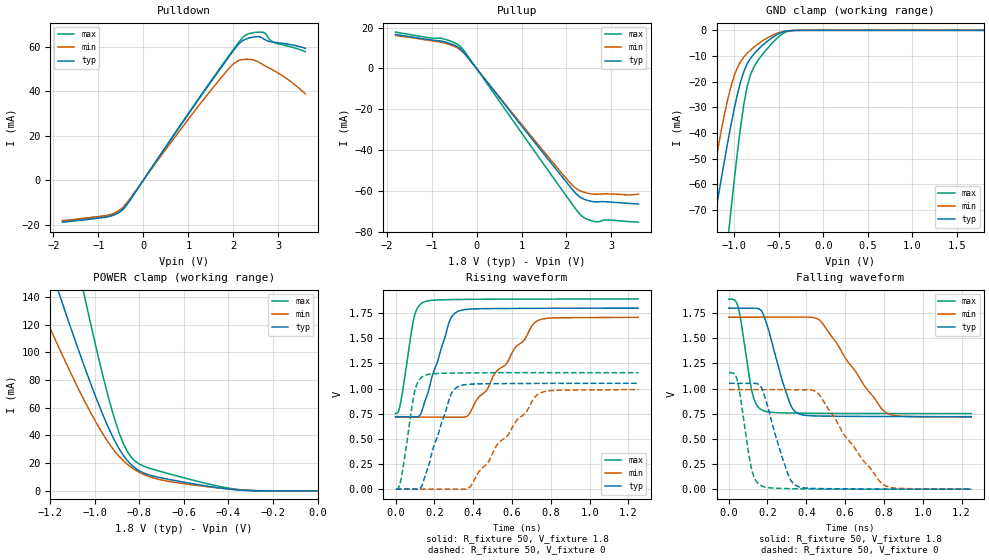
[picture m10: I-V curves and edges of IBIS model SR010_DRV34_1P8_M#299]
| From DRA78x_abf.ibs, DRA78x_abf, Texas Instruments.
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| Model based on original model for DDR_DIFFIOPB_V
|   Sub model SR010_DRV34_1P8
[model]   SR010_DRV34_1P8_M#299
|[Description]  [1.8V-I/O-X-X]
|   , ,
|[Input Load]
|[Output Drive]
|Voltage   1.8V
|Mode   I/O
Model_type   I/O
Polarity   Non-Inverting
Enable   Active-Low
Vinl =  0.775
Vinh =  1.025
Cref =  15.0000pF
Rref =  100.0000M
Vref =  0V
Vmeas =  0.9
C_comp   2p   2p   2p
[Model Spec]
Vinl   0.78   0.735   0.825
Vinh   1.02   0.975   1.065
[Receiver Thresholds]
Tslew_ac = 0.5n
Vth = 0.9
Vth_max = 0.945
Vth_min = 0.81
Vinh_ac = 0.2
Vinh_dc = 0.125
Vinl_ac = -0.2
Vinl_dc = -0.125
[Temperature Range]   25   125   -40
[Voltage Range]   1.8   1.71   1.89
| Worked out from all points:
|   slope of the pulldown table from 0 to 0.27 V, typ, clamps not added: 33.3 ohm
|   slope of the pullup table from 0 to 0.27 V, typ, clamps not added: 35.5 ohm
|   GND clamp passes 1 mA (typ) near -0.48 V on its own axis
|   POWER clamp passes 1 mA (typ) near -0.38 V on its own axis
|   rising waveform, R_fixture 50, V_fixture 1.8: 20-80 % time 101ps typ, 243ps min, 53.2ps max; typ from 0.721 V to 1.8 V
|   rising waveform, R_fixture 50, V_fixture 0: 20-80 % time 101ps typ, 241ps min, 53.2ps max; typ from 0 V to 1.05 V
|   falling waveform, R_fixture 50, V_fixture 1.8: 20-80 % time 94.6ps typ, 214ps min, 55.3ps max; typ from 1.8 V to 0.721 V
|   falling waveform, R_fixture 50, V_fixture 0: 20-80 % time 96.6ps typ, 219ps min, 54.7ps max; typ from 1.05 V to 0 V
[POWER_clamp]
-1.8V     464.6mA    344.4mA    740.8mA
-1.273V   197mA      143.3mA    314.4mA
-1.164V   144mA      104.2mA    229mA
-1.145V   135.3mA    97.86mA    215mA
-1.055V   93.25mA    67.59mA    146.5mA
-1.036V   85.18mA    61.89mA    133.3mA
-909.1mV  35.72mA    28.41mA    50.73mA
-872.7mV  25.87mA    21.94mA    34.5mA
-818.2mV  16.45mA    15.08mA    21.33mA
-690.9mV  9.084mA    7.592mA    13.42mA
-400mV    1.38mA     1.43mA     2.039mA
0V        227.3nA    761nA      1.176uA
[Pulldown]
-1.8V     -18.96mA   -18.25mA   -18.29mA
-818.2mV  -16.64mA   -15.93mA   -16.11mA
-600mV    -15.26mA   -14.42mA   -14.86mA
-436.4mV  -12.77mA   -11.85mA   -12.76mA
1.255V    37.14mA    34.14mA    37.53mA
1.855V    54.25mA    49.2mA     54.74mA
2.073V    60.22mA    53.41mA    60.8mA
2.291V    63.64mA    54.44mA    65.5mA
2.618V    64.32mA    52.48mA    66.68mA
2.727V    62.98mA    51.19mA    65.69mA
2.891V    62.13mA    49.45mA    62.08mA
3.6V      59.37mA    38.9mA     57.88mA
[Pullup]
-1.8V     16.66mA    16.14mA    17.84mA
-1.036V   14.05mA    13.69mA    15mA
-763.6mV  13.33mA    12.72mA    14.68mA
-490.9mV  11.4mA     10.78mA    12.65mA
-327.3mV  8.923mA    8.488mA    10.05mA
2.018V    -56.27mA   -54.56mA   -63.19mA
2.182V    -60.67mA   -58.29mA   -68.22mA
2.345V    -63.65mA   -60.35mA   -72.46mA
2.509V    -64.94mA   -61.33mA   -74.33mA
2.673V    -65.44mA   -61.69mA   -75.21mA
2.891V    -65.36mA   -61.45mA   -74.26mA
3.6V      -66.47mA   -61.61mA   -75.37mA
[GND_clamp]
-1.8V     -200.8mA   -187.9mA   -345.9mA
-1.327V   -95.75mA   -76.22mA   -171.1mA
-1.255V   -80.19mA   -60.47mA   -144.9mA
-1.218V   -72.53mA   -52.92mA   -131.9mA
-1.073V   -43.32mA   -26.59mA   -81.54mA
-1.036V   -36.61mA   -21.6mA    -69.55mA
-963.6mV  -24.61mA   -14.37mA   -47.01mA
-854.5mV  -12.98mA   -8.864mA   -21.66mA
-781.8mV  -9.263mA   -6.573mA   -14.36mA
-672.7mV  -5.498mA   -3.827mA   -8.897mA
-345.5mV  -48.81uA   -73.08uA   -79.37uA
1.8V      227.3nA    3.986uA    988nA
[Ramp]
dV/dt_f   0.647957/94.640072p 0.59676242/0.21402689n  0.6831801/55.297889p
dV/dt_r 0.63285444/0.10159097n 0.59531046/0.24136669n  0.6962006/53.228439p
R_load = 50
[Rising Waveform]
R_fixture = 50
V_fixture = 1.8
V_fixture_min = 1.71
V_fixture_max = 1.89
0s        720.8mV    716.7mV    752.8mV
25.2ps    720.4mV    716.6mV    852.1mV
95.22ps   720mV      716.6mV    1.707V
125ps     732.3mV    716.6mV    1.832V
144.3ps   832.3mV    716.6mV    1.859V
275.5ps   1.657V     716.5mV    1.884V
320.9ps   1.767V     715.4mV    1.886V
377.2ps   1.79V      740.6mV    1.887V
729.5ps   1.798V     1.672V     1.89V
1.25ns    1.8V       1.71V      1.89V
[Rising Waveform]
R_fixture = 50
V_fixture = 0
V_fixture_min = 0
V_fixture_max = 0
1.723ps   0V         0V         0V
32.03ps   0V         0V         138.9mV
98.8ps    0V         0V         974.3mV
146.1ps   96.14mV    0V         1.127V
278.8ps   911.3mV    0V         1.154V
324.6ps   1.021V     0V         1.155V
384.9ps   1.044V     25.07mV    1.156V
524.2ps   1.049V     443.6mV    1.158V
740.7ps   1.051V     950.9mV    1.158V
1.252ns   1.053V     990.1mV    1.159V
[Falling Waveform]
R_fixture = 50
V_fixture = 1.8
V_fixture_min = 1.71
V_fixture_max = 1.89
0s        1.8V       1.71V      1.89V
46.31ps   1.8V       1.71V      1.826V
122.2ps   1.8V       1.71V      953.1mV
143.2ps   1.799V     1.71V      840.5mV
173.4ps   1.76V      1.71V      784.7mV
309ps     884.6mV    1.71V      757.5mV
356.5ps   753.8mV    1.71V      756mV
476.3ps   726.9mV    1.666V     753.8mV
812.5ps   722.3mV    759.6mV    752mV
1.25ns    720.8mV    716.7mV    751.8mV
[Falling Waveform]
R_fixture = 50
V_fixture = 0
V_fixture_min = 0
V_fixture_max = 0
1.723ps   1.053V     990.1mV    1.159V
42.83ps   1.053V     990.1mV    1.092V
117.2ps   1.053V     990.1mV    207.3mV
169ps     1.009V     990.1mV    32.57mV
303.8ps   159.5mV    990mV      5.25mV
351.1ps   31.61mV    989.9mV    3.57mV
462.9ps   5.934mV    947.6mV    0V
597.1ps   2.967mV    534.7mV    0V
801.7ps   0V         39.38mV    0V
1.252ns   0V         0V         0V
